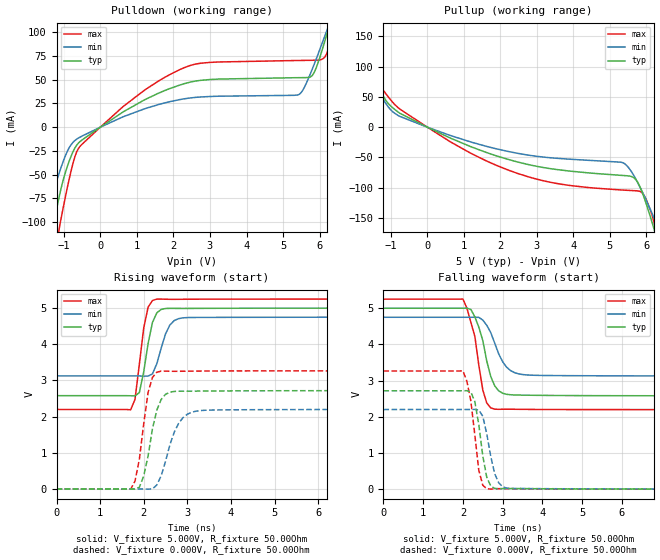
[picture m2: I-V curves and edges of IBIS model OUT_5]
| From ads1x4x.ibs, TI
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|   Output 5.0V Model
[Model]   OUT_5
Model_type   Output
|Signals   nDRDY
| variable   typ   min   max
|C_comp Output average
C_comp   9.568pF   6.828pF   15.724pF
|C_comp Output Low
|C_comp   3.599pF   4.364pF   2.907pF
|C_comp Output High
|C_comp   15.536pF   9.291pF   28.541pF
[Model Spec]
|Timing spec test load voltage corners 0.45*VCC
Vmeas   1.5V   1.35V   1.65V
Vref   1.5V   1.35V   1.65V
|Junction Temperature
[Temperature Range]   40.0   105.0   -40.0
[Voltage range]   5.0V   4.75V   5.25V
[pullup reference]   5.0V   4.75V   5.25V
[power clamp reference]   5.0V   4.75V   5.25V
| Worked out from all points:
|   slope of the pulldown table from 0 to 0.75 V, typ, clamps not added: 39.8 ohm
|   slope of the pullup table from 0 to 0.75 V, typ, clamps not added: 35.7 ohm
|   falling waveform, V_fixture 5.000V, R_fixture 50.00Ohm: 20-80 % time 333ps typ, 394ps min, 297ps max; typ from 5 V to 2.58 V
|   rising waveform, V_fixture 5.000V, R_fixture 50.00Ohm: 20-80 % time 216ps typ, 260ps min, 199ps max; typ from 2.58 V to 5 V
|   rising waveform, V_fixture 0.000V, R_fixture 50.00Ohm: 20-80 % time 266ps typ, 359ps min, 221ps max; typ from 0 V to 2.72 V
|   falling waveform, V_fixture 0.000V, R_fixture 50.00Ohm: 20-80 % time 225ps typ, 245ps min, 219ps max; typ from 2.72 V to 0 V
[Pulldown]
|   Voltage   I(typ)   I(min)   I(max)
-5V       -958.8mA   -692.3mA   -1.337A
-1.6V     -169.2mA   -111.5mA   -245.6mA
-1.3V     -106.2mA   -69.87mA   -153.1mA
-1.15V    -77.41mA   -51.06mA   -112.3mA
-850mV    -35.45mA   -21.4mA    -54.17mA
-550mV    -14.95mA   -10.38mA   -19.9mA
2.45V     47.36mA    30.72mA    64.88mA
5.45V     52.13mA    34.7mA     70.25mA
5.85V     57.37mA    65.99mA    70.5mA
6.25V     104.7mA    107mA      84.1mA
6.4V      124.5mA    121.9mA    108.6mA
10V       368.7mA    314.6mA    437.8mA
[Pullup]
|   Voltage   I(typ)   I(min)   I(max)
-5V       290.3mA    256mA      340.9mA
-2.65V    190.9mA    164.9mA    225.4mA
-2.3V     166.6mA    142.8mA    198.1mA
-2V       140.9mA    120.1mA    168.1mA
-1.2V     50.74mA    44.99mA    60.61mA
0V        434.7pA    425pA      331pA
2.5V      -57.89mA   -43.47mA   -76.86mA
5.35V     -79.71mA   -58.6mA    -103.8mA
5.75V     -89.85mA   -90.26mA   -105.1mA
6.2V      -166.3mA   -148.8mA   -154.9mA
6.35V     -197.5mA   -170.7mA   -195.7mA
10V       -1.05A     -803.8mA   -1.37A
[Ramp]
R_load = 50.00Ohm
|   typ   min   max
dV/dt_r   1.631V/265.988ps   1.320V/358.938ps   1.959V/221.292ps
dV/dt_f   1.452V/333.285ps 973.923mV/394.292ps   1.831V/297.388ps
[Falling Waveform]
V_fixture = 5.000V
V_fixture_min = 4.750V
V_fixture_max = 5.250V
R_fixture = 50.00Ohm
|   Time   V(typ)   V(min)   V(max)
0s        5V         4.75V      5.25V
2ns       5V         4.75V      5.253V
2.2ns     4.967V     4.75V      4.61V
2.3ns     4.762V     4.751V     4.224V
2.5ns     4.106V     4.673V     2.74V
2.6ns     3.538V     4.528V     2.381V
2.8ns     2.855V     4.033V     2.21V
3.1ns     2.621V     3.37V      2.21V
3.5ns     2.598V     3.167V     2.205V
10ns      2.58V      3.127V     2.198V
[Rising Waveform]
V_fixture = 5.000V
V_fixture_min = 4.750V
V_fixture_max = 5.250V
R_fixture = 50.00Ohm
|   Time   V(typ)   V(min)   V(max)
0s        2.58V      3.127V     2.198V
1.7ns     2.577V     3.127V     2.189V
1.8ns     2.572V     3.126V     2.479V
1.9ns     2.667V     3.125V     3.453V
2ns       3.243V     3.12V      4.454V
2.1ns     4.022V     3.122V     5.025V
2.3ns     4.87V      3.463V     5.25V
2.6ns     4.994V     4.535V     5.244V
2.9ns     4.992V     4.731V     5.245V
10ns      5V         4.75V      5.25V
[Rising Waveform]
V_fixture = 0.000V
V_fixture_min = 0.000V
V_fixture_max = 0.000V
R_fixture = 50.00Ohm
|   Time   V(typ)   V(min)   V(max)
0s        1.244nV    1.436nV    1.191nV
1.7ns     -372.6uV   84.53uV    -5.649mV
1.8ns     -4.336mV   182.2uV    216.3mV
2ns       361.8mV    -403uV     1.806V
2.1ns     913.8mV    -4.85mV    2.67V
2.3ns     2.18V      110mV      3.227V
2.5ns     2.618V     763.1mV    3.259V
2.8ns     2.702V     1.814V     3.254V
3.2ns     2.705V     2.151V     3.259V
10ns      2.718V     2.2V       3.265V
[Falling Waveform]
V_fixture = 0.000V
V_fixture_min = 0.000V
V_fixture_max = 0.000V
R_fixture = 50.00Ohm
|   Time   V(typ)   V(min)   V(max)
0s        2.718V     2.2V       3.265V
2ns       2.719V     2.2V       3.269V
2.2ns     2.685V     2.202V     2.433V
2.3ns     2.415V     2.205V     1.494V
2.4ns     1.78V      2.187V     519.2mV
2.5ns     915.7mV    2.016V     109.2mV
2.6ns     326.7mV    1.527V     8.727mV
2.8ns     21.48mV    425.9mV    10.02mV
3.1ns     18.14mV    29.03mV    12.52mV
10ns      1.244nV    1.436nV    1.191nV
